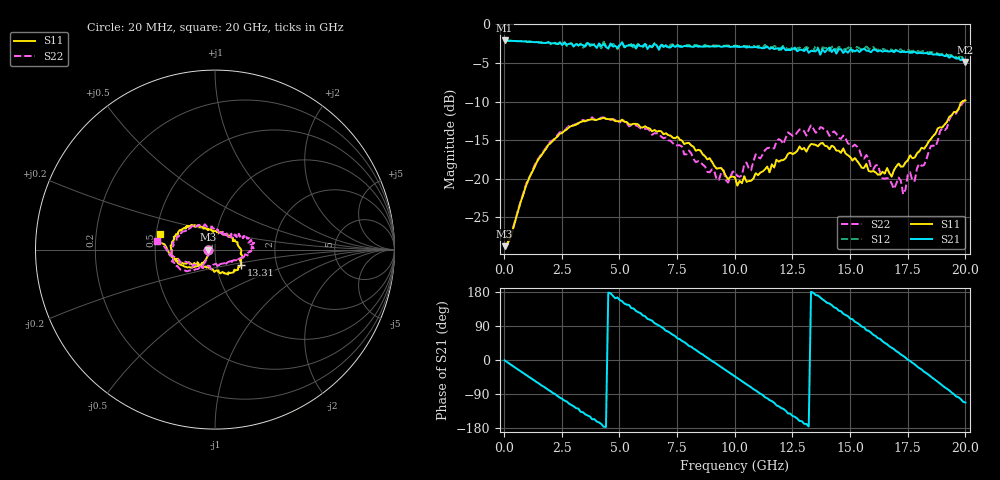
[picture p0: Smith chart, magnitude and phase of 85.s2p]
!Agilent Technologies,N5230A,US43500223,A.07.50.48
!Agilent N5230A: A.07.50.48
!Date: Tuesday, September 15, 2015 19:50:29
!Correction: S11(Full 2 Port(1,2))
!S21(Full 2 Port(1,2))
!S12(Full 2 Port(1,2))
!S22(Full 2 Port(1,2))
!S2P File: Measurements: S11, S21, S12, S22:
# Hz S  dB  R 50
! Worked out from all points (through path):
!   201 points, 20 MHz to 20 GHz, reference 50 ohm
!   highest |S21| = -2.08 dB at 20 MHz (marker M1); lowest = -4.9 dB at 20 GHz (marker M2)
!   group delay of S21, straight-line fit = 114 ps
!   lowest |S11| = -28.8 dB at 20 MHz (marker M3), VSWR 1.08, Z = 46.5 - j0.0273 ohm
!   |S11| at or under -10 dB: start of sweep to 19.87 GHz
!   |S22| runs from -28.7 to -9.8 dB; largest |S21 - S12| = 0.079
!   S11 on the Smith chart (normalised r, x): 20 MHz: 0.93, -0.00; 13.31 GHz: 1.32, -0.23; 20 GHz: 0.52, +0.10
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2e7  -28.75 -179.5  -2.08 -0.9  -2.08 -0.9  -28.69 -179.4
9.191e8  -21.16 -132.0  -2.19 -38.2  -2.20 -38.2  -20.98 -128.0
1.9181e9  -15.60 -142.8  -2.31 -78.9  -2.30 -79.0  -15.48 -135.5
3.4166e9  -12.55 -168.8  -2.68 -137.8  -3.02 -137.1  -12.38 -157.5
4.3157e9  -12.09 174.8  -2.55 -176.3  -2.25 -173.1  -12.06 -173.3
5.1149e9  -12.34 162.9  -2.31 155.0  -2.37 155.1  -12.42 171.4
6.7133e9  -13.81 139.1  -3.28 90.7  -3.17 91.5  -14.19 142.2
7.5125e9  -14.52 133.7  -2.75 57.1  -2.66 60.3  -15.67 123.3
8.7113e9  -17.10 118.7  -2.87 9.8  -2.64 11.1  -18.41 95.2
1.001e10  -19.82 85.4  -2.87 -43.3  -2.75 -42.3  -19.10 53.7
1.14086e10  -18.43 33.6  -2.87 -100.9  -2.96 -100.8  -16.03 29.2
1.25075e10  -16.81 -8.7  -3.21 -147.8  -2.94 -146.5  -14.45 21.4
1.33067e10  -15.51 -29.9  -3.41 179.9  -3.38 -176.5  -13.08 9.6
1.34066e10  -15.55 -35.2  -3.47 177.5  -3.46 -178.8  -13.50 8.0
1.41059e10  -16.18 -45.8  -2.99 149.1  -3.46 151.2  -14.45 -2.9
1.5005e10  -17.19 -69.1  -3.27 108.8  -2.78 110.3  -15.58 -13.1
1.56044e10  -18.60 -87.6  -3.14 86.2  -3.19 86.6  -17.41 -24.0
1.67033e10  -19.26 -127.6  -3.52 36.1  -3.13 37.8  -20.06 -52.6
1.73027e10  -18.42 -144.7  -3.51 10.8  -3.54 11.7  -22.01 -86.6
1.82018e10  -16.13 -151.1  -3.74 -30.7  -3.38 -29.3  -18.26 -129.5
1.91009e10  -12.99 -166.4  -4.12 -72.0  -3.70 -70.2  -13.71 -161.9
2e10  -9.86 164.0  -4.86 -112.2  -4.74 -112.4  -9.76 172.0
